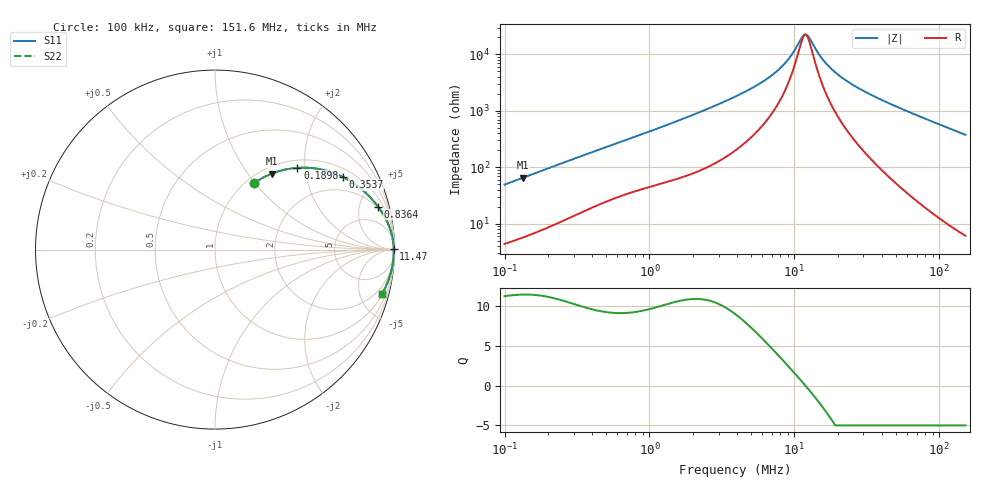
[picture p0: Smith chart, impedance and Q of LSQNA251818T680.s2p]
! LSQNA251818T680  S-PARAMETER MODEL  ( General Type )
! Model Generated by TAIYO YUDEN Corporation (http://www.ty-top.com)
! Version 2.0
! TAIYO YUDEN Control No. 100810NF25SB-FKC
! Copyright(c) 2007 TAIYO YUDEN CO.,LTD. All Rights Reserved.
! Product Description (link to TY-COMPAS)
! https://ds.yuden.co.jp/TYCOMPAS/or/detail?pn=LSQNA251818T680K&u=M
! Products Name : Inductors
! Characteristics :
!  Inductance : 68 uH , SRF(min) : 9.5 MHz , DC Resistance(max) : 1.95 Ohm
!  Rated Current : Saturation :70 mA , Temp Rise : 310 mA (40 degC)
!  Case Size : 2.5 x 1.8 / 0.098 x 0.071 [mm/inch] , Thickness : 1.8 / 0.071 [mm/inch]
!  (Conditions: Temperature = 25 degC , DC Bias Current/Voltage = 0A / 0V)
! External Node Assignments :
!  1  o---GGG---o  2
! GND o---------o GND
! Frequency Range : 0.1MHz  -  151.640846MHz  [ 402 STEP ]
# MHz S RI R 50
! Freq[MHz].  S11 Real  S11 Imag  S21 Real  S21 Imag  S12 Real  S12 Imag  S22 Real  S22 Imag
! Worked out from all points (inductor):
!   401 points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, 100 kHz to 151.6 MHz, reference 50 ohm
!   read as one part in series: L = 77.7 uH near 103.7 kHz
!   highest Q = 11.4 at 134 kHz (marker M1), where L = 77.6 uH
!   self-resonance near 11.9 MHz
!   S11 on the Smith chart (normalised r, x): 100 kHz: 1.09, +0.99; 189.8 kHz: 1.16, +1.82; 353.7 kHz: 1.33, +3.29; 836.4 kHz: 1.78, +7.27; 11.47 MHz: open; 151.6 MHz: 1.12, -7.55
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0.1  0.2168 0.3698  0.7832 -0.3698  0.7832 -0.3698  0.2168 0.3698
0.134039  0.3154 0.4229  0.6846 -0.4229  0.6846 -0.4229  0.3154 0.4229
0.189811  0.4596 0.4557  0.5404 -0.4557  0.5404 -0.4557  0.4596 0.4557
0.341025  0.7 0.4106  0.3 -0.4106  0.3 -0.4106  0.7 0.4106
0.353745  0.7126 0.4045  0.2874 -0.4045  0.2874 -0.4045  0.7126 0.4045
0.529219  0.8266 0.3279  0.1734 -0.3279  0.1734 -0.3279  0.8266 0.3279
0.836444  0.9081 0.24  0.0919 -0.24  0.0919 -0.24  0.9081 0.24
1.162983  0.9441 0.1847  0.0559 -0.1847  0.0559 -0.1847  0.9441 0.1847
3.894109  0.9908 0.0549  0.00922 -0.0549  0.00922 -0.0549  0.9908 0.0549
5.825765  0.9938 0.0315  0.00617 -0.0315  0.00617 -0.0315  0.9938 0.0315
7.667144  0.9949 0.0185  0.00514 -0.0185  0.00514 -0.0185  0.9949 0.0185
9.20776  0.9953 0.0106  0.00472 -0.0106  0.00472 -0.0106  0.9953 0.0106
11.4704  0.9956 0.00156  0.00444 -0.00156  0.00444 -0.00156  0.9956 0.00156
11.89824  0.9956 6.53e-05  0.00441 -6.53e-05  0.00441 -6.53e-05  0.9956 6.53e-05
12.34203  0.9956 -0.00143  0.00438 0.00143  0.00438 0.00143  0.9956 -0.00143
13.2799  0.9957 -0.00443  0.00435 0.00443  0.00435 0.00443  0.9957 -0.00443
15.94833  0.9957 -0.0121  0.00435 0.0121  0.00435 0.0121  0.9957 -0.0121
20.23447  0.9954 -0.0227  0.00456 0.0227  0.00456 0.0227  0.9954 -0.0227
28.1338  0.9946 -0.0398  0.00542 0.0398  0.00542 0.0398  0.9946 -0.0398
45.28783  0.991 -0.0728  0.00896 0.0728  0.00896 0.0728  0.991 -0.0728
84.40164  0.9759 -0.1412  0.0241 0.1412  0.0241 0.1412  0.9759 -0.1412
151.6408  0.9309 -0.2456  0.0691 0.2456  0.0691 0.2456  0.9309 -0.2456
